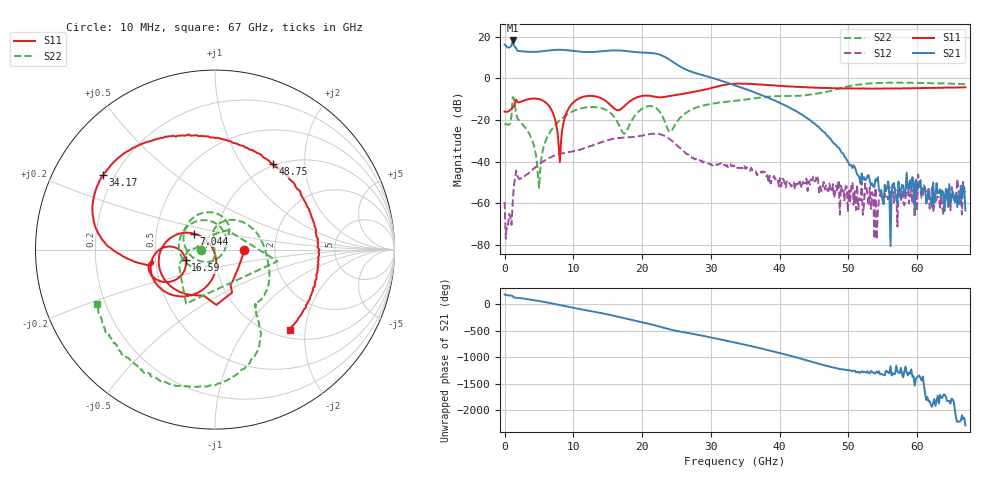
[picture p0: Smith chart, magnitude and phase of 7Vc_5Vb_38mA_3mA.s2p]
! MARKI MICROWAVE INC.
! Date:  05/05/2020
! Model Number:  APM-7099CH
! Description:  2-port Small Signal S-parameter data for APM-7099CH
! Frequency Range:  10 MHz to 67 GHz
! Port Configuration:  PORT 1: Input
!  PORT 2: Output
! Bias Condition: Vc = +7V, Vb = +5V
! APM-7099CH s2p files are only valid for small signal conditions (below -5 dBm input power)
!S2P File: Measurements: Mag<S11> Ang<S11>, Mag<S21> Ang<S21>, Mag<S12> Ang<S12>, Mag<S22> Ang<S22>!row 1
# Hz S  dB  R 50
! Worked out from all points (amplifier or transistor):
!   401 points, 10 MHz to 67 GHz, reference 50 ohm
!   highest |S21| = 18.3 dB at 1.182 GHz (marker M1)
!   |S21| within 3 dB of that: 876 MHz to 1.501 GHz (624.8 MHz wide, 52.6 % of centre)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
!   unconditionally stable (mu >= 1): start of sweep to end of sweep
!   at 11.06 GHz: K = 4.98, MAG = 13.6 dB, |S12| = -34.1 dB
!   at 33.51 GHz: K = 37.51, MAG = 0.5 dB, |S12| = -41.9 dB
!   at 67 GHz: K = 138640.70, MAG = -58.3 dB, |S12| = -55.8 dB
!   S11 on the Smith chart (normalised r, x): 10 MHz: 1.38, -0.01; 7.044 GHz: 0.78, +0.14; 16.59 GHz: 0.71, -0.09; 34.17 GHz: 0.16, +0.30; 48.75 GHz: 0.98, +1.39; 67 GHz: 1.16, -1.66
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1e7  -15.98 -0.8  16.27 178.8  -59.44 65.4  -22.32 -178.1
1.182325e9  -13.82 -61.3  18.25 149.7  -60.11 88.4  -9.01 -10.5
1.68475e9  -10.22 -88.6  14.40 115.5  -44.30 -79.7  -17.00 178.8
4.36435e9  -9.68 -156.4  12.77 70.9  -43.17 -161.0  -33.38 122.4
7.04395e9  -16.71 142.4  13.63 7.8  -37.44 136.3  -23.77 -102.6
9.221125e9  -15.06 -97.2  13.52 -51.2  -35.53 87.5  -17.10 -132.9
1.123082e10  -9.04 -135.2  12.82 -101.2  -33.99 51.9  -14.33 -169.4
1.441285e10  -10.17 -179.8  13.13 -178.8  -30.36 -11.9  -14.64 120.1
1.659002e10  -15.22 -160.3  13.45 118.6  -28.66 -65.1  -22.05 36.6
1.80973e10  -11.32 -142.4  13.00 74.2  -28.32 -102.0  -22.82 -112.3
1.993952e10  -8.47 -156.1  12.45 20.9  -27.58 -145.7  -14.72 162.6
2.127932e10  -8.46 -167.1  12.22 -21.2  -26.68 176.9  -13.31 110.5
2.245165e10  -9.08 -168.7  11.53 -62.3  -26.71 137.0  -15.58 65.1
2.379145e10  -8.59 -166.4  9.42 -109.5  -28.70 90.4  -24.92 55.1
2.513125e10  -7.86 -168.4  6.49 -148.4  -32.38 53.7  -20.60 95.9
2.898318e10  -5.54 -177.1  1.40 118.8  -40.06 6.6  -12.98 39.8
3.3505e10  -2.55 152.1  -3.34 -4.7  -41.92 -42.5  -10.74 -5.9
3.41749e10  -2.50 146.4  -4.11 -23.5  -42.96 -49.1  -10.55 -10.9
4.472582e10  -4.39 79.0  -20.99 -7.8  -48.90 14.1  -7.65 -56.6
4.874522e10  -4.80 55.6  -34.05 -144.3  -65.51 -16.7  -4.75 -64.6
5.594665e10  -4.82 11.3  -54.98 140.3  -52.11 -97.9  -2.06 -106.8
6.7e10  -4.27 -46.9  -63.53 -124.7  -55.84 -176.5  -2.81 -155.1
